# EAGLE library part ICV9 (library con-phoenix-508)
PHOENIX
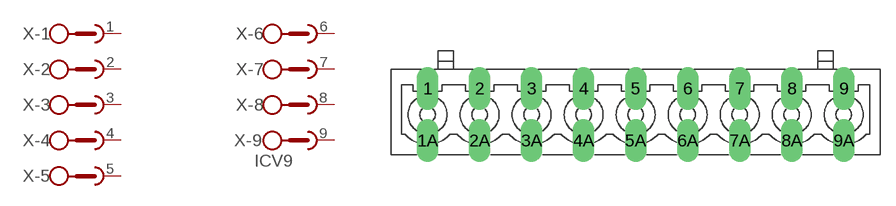
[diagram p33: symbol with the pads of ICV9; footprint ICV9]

Designator prefix X; gates -1=SKB -2=SKB -3=SKB -4=SKB -5=SKB -6=SKB -7=SKB -8=SKB -9=SKBV

## ICV9 (OC_FARNELL: unknown; OC_NEWARK: unknown)  [ICV9]
1  -1:1  pas
2  -2:1  pas
3  -3:1  pas
4  -4:1  pas
5  -5:1  pas
6  -6:1  pas
7  -7:1  pas
8  -8:1  pas
9  -9:1  pas

## Footprint ICV9 (pad centres in mm)
PHOENIX
drill 1.397 long: 1 -20.32,2.54; 1A -20.32,-2.54; 2 -15.24,2.54; 2A -15.24,-2.54; 3 -10.16,2.54; 3A -10.16,-2.54; 4 -5.08,2.54; 4A -5.08,-2.54; 5 0,2.54; 5A 0,-2.54; 6 5.08,2.54; 6A 5.08,-2.54; 7 10.16,2.54; 7A 10.16,-2.54; 8 15.24,2.54; 8A 15.24,-2.54; 9 20.32,2.54; 9A 20.32,-2.54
